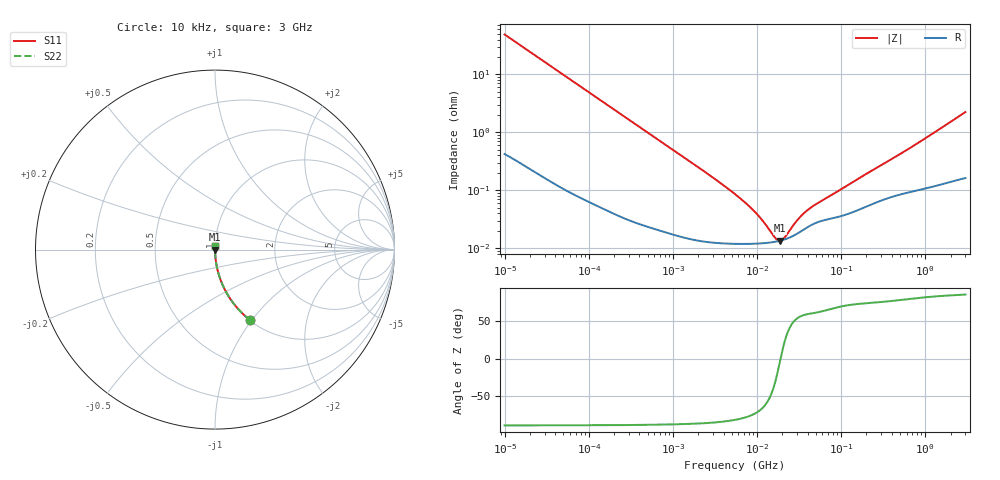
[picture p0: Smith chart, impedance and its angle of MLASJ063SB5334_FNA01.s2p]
! MLASJ063SB5334_FNA01  S-PARAMETER MODEL  ( Standard Model )
! Model Generated by TAIYO YUDEN Corporation (http://www.ty-top.com)
! Version 1.0
! TAIYO YUDEN Control No. 220601
! Copyright(c) 2014 TAIYO YUDEN CO.,LTD. All Rights Reserved.
! Product Description (link to TY-COMPAS)
! https://ds.yuden.co.jp/TYCOMPAS/or/detail?pn=MLASJ063SB5334MFNA01&u=M
! Products Name : Multilayer Ceramic Capacitors
! Characteristics :
!  Capacitance : 0.33 [uF] , Rated Voltage : 6.3 [V] , TCC : X5R
!  Case Size : 0.6 x 0.3 / 0.024 x 0.012 [mm/inch] , Thickness : 0.3 / 0.012 [mm/inch]
!  (Conditions: Temperature = 25 [degC] , DC Bias Voltage = 0 [V])
! External Node Assignments :
!  1  o---| |---o  2
! GND o---------o GND
! Frequency Range : 10kHz  -  3GHz  [ 401 STEP ]
# MHZ S RI R 50
! Freq[MHz].  S11 Real  S11 Imag  S21 Real  S21 Imag  S12 Real  S12 Imag  S22 Real  S22 Imag
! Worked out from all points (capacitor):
!   401 points, 10 kHz to 3 GHz, reference 50 ohm
!   read as one part in series: C = 325 nF near 10.65 kHz
!   lowest |Z| = 13.5 mohm at 18.73 MHz (marker M1)
!   series resonance near 19.06 MHz, so ESL is about 210 pH
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0.01  0.1947 -0.3917  0.8053 0.3917  0.8053 0.3917  0.1947 -0.3917
0.015066  0.0977 -0.2924  0.9023 0.2924  0.9023 0.2924  0.0977 -0.2924
0.022699  0.0465 -0.2058  0.9535 0.2058  0.9535 0.2058  0.0465 -0.2058
0.041322  0.0152 -0.1173  0.9848 0.1173  0.9848 0.1173  0.0152 -0.1173
0.082683  0.00428 -0.0595  0.9957 0.0595  0.9957 0.0595  0.00428 -0.0595
0.199902  0.00101 -0.0249  0.999 0.0249  0.999 0.0249  0.00101 -0.0249
0.683653  0.000258 -0.00734  0.9997 0.00734  0.9997 0.00734  0.000258 -0.00734
2.570001  0.000132 -0.00194  0.9999 0.00194  0.9999 0.00194  0.000132 -0.00194
5.477226  0.00012 -0.000853  0.9999 0.000853  0.9999 0.000853  0.00012 -0.000853
9.361346  0.00012 -0.000413  0.9999 0.000413  0.9999 0.000413  0.00012 -0.000413
11.67315  0.000122 -0.000273  0.9999 0.000273  0.9999 0.000273  0.000122 -0.000273
16.51234  0.00013 -7.71e-05  0.9999 7.71e-05  0.9999 7.71e-05  0.00013 -7.71e-05
17.5871  0.000132 -4.31e-05  0.9999 4.31e-05  0.9999 4.31e-05  0.000132 -4.31e-05
18.73182  0.000135 -9.18e-06  0.9999 9.18e-06  0.9999 9.18e-06  0.000135 -9.18e-06
19.95104  0.000138 2.46e-05  0.9999 -2.46e-05  0.9999 -2.46e-05  0.000138 2.46e-05
21.24962  0.000142 5.84e-05  0.9999 -5.84e-05  0.9999 -5.84e-05  0.000142 5.84e-05
28.22191  0.00017 0.000212  0.9998 -0.000212  0.9998 -0.000212  0.00017 0.000212
33.04079  0.000195 0.000296  0.9998 -0.000296  0.9998 -0.000296  0.000195 0.000296
45.28751  0.000256 0.000456  0.9997 -0.000456  0.9997 -0.000456  0.000256 0.000456
374.4521  0.000755 0.00319  0.9992 -0.00319  0.9992 -0.00319  0.000755 0.00319
773.2692  0.00102 0.00612  0.999 -0.00612  0.999 -0.00612  0.00102 0.00612
3000  0.00212 0.0222  0.9979 -0.0222  0.9979 -0.0222  0.00212 0.0222
